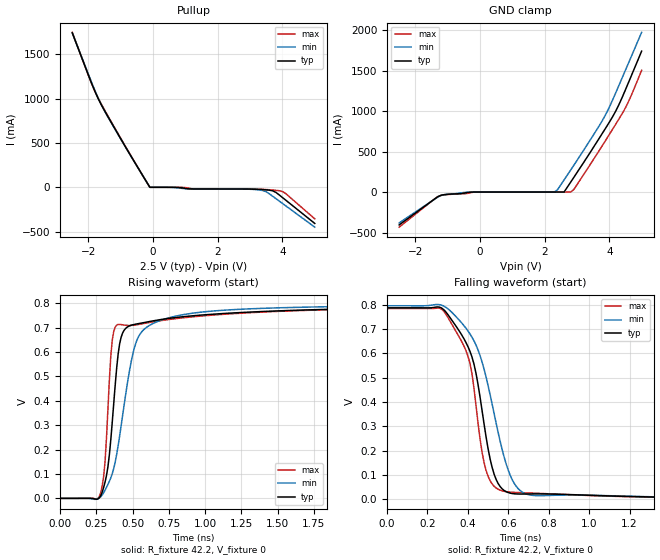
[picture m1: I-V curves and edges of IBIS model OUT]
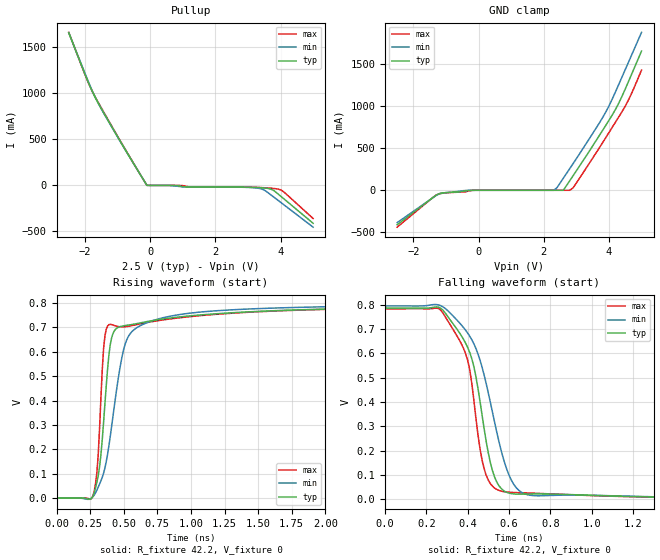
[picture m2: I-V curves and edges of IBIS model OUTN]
|   IBIS File of SG2520HHN D
|   HCSL Zdiff=85, Vcc=2.5V, fo>212.5MHz
[IBIS Ver]   3.2
[File Name]   sg2520hhn_hf_85_25v.ibs
[File Rev]   1.0
[Date]   Aug. 4, 2020
[Source]
[Notes]
Created by Minoru Kozaki
[Disclaimer]
Seiko Epson Corporation makes no warranty with respect to the
information contained herein.
[Copyright]
Copyright(C) 2020, Seiko Epson Corporation. All rights reserved.
|   Component
[Component]   SG2520HHN
[Manufacturer]  Seiko Epson Corporation
[Package]
R_pkg   17.7m   NA   NA
L_pkg   235p   NA   NA
C_pkg   208f   NA   NA
[Pin]   signal_name   model_name   R_pin   L_pin   C_pin
1   OE/ST   NC
2   NC   NC
3   GND   GND
4   OUT   OUT   17.7m   235p   208f
5   OUTN   OUTN   10.4m   129p   221f
6   VCC   POWER
[Diff Pin] inv_pin  vdiff  tdelay_typ
4   5   0   0
| Models and submodels in the file (2): OUT (Open_source), OUTN (Open_source)
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|   Model OUT
[Model]   OUT
Model_type   Open_source
Polarity   Non-Inverting
Vref = 0
Vmeas = 0.4
Rref = 42.2
Cref = 0
C_comp   12.0p   12.0p   12.0p
[Temperature Range]   25   105   -40
[Voltage Range]   2.5   2.25   2.75
[Pullup Reference]   2.5   2.25   2.75
[GND Clamp Reference]   0   0   0
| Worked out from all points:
|   GND clamp passes 1 mA (typ) near -0.25 V on its own axis
|   falling waveform, R_fixture 42.2, V_fixture 0: 20-80 % time 113ps typ, 146ps min, 96.9ps max; typ from 0.787 V to 0 V
|   rising waveform, R_fixture 42.2, V_fixture 0: 20-80 % time 74ps typ, 139ps min, 45.8ps max; typ from 0 V to 0.786 V
[Pullup]
-2.5V     1.74A      1.738A     1.746A
-1.9V     1.169A     1.18A      1.166A
-1.7V     1A         1.006A     1.004A
-1.3V     734.6mA    730.6mA    742.7mA
-100mV    31.32uA    15.33uA    89.15uA
700mV     -480.9uA   -4.431mA   -3.81uA
1.1V      -17.61mA   -18.31mA   -9.992mA
2.9V      -19.54mA   -20.86mA   -19.1mA
3.4V      -25.62mA   -36.48mA   -23.79mA
3.7V      -39.9mA    -101.2mA   -30.43mA
4V        -114.7mA   -181.3mA   -47.79mA
5V        -407mA     -448.8mA   -355mA
[GND Clamp]
-2.5V     -405.6mA   -380.9mA   -433.4mA
-1.2V     -39.03mA   -41.71mA   -40.52mA
-100mV    -21.28uA   -12.94uA   -96.75uA
2.3V      -1.475uA   3.582uA    -3.007uA
2.4V      -1.333uA   29.72mA    -2.745uA
2.6V      31.32uA    149mA      -2.258uA
2.8V      119.4mA    268.7mA    13.29uA
2.9V      179.5mA    328.8mA    29.86mA
3.8V      734.6mA    893.4mA    583.2mA
4.2V      1A         1.226A     838.7mA
4.6V      1.358A     1.598A     1.122A
5V        1.74A      1.972A     1.502A
[Falling Waveform]
R_fixture = 42.2
V_fixture = 0
V_fixture_min = 0
V_fixture_max = 0
0s        786.9mV    795.4mV    783.9mV
270ps     786.1mV    797.8mV    781.5mV
400ps     628.6mV    692.7mV    589.6mV
440ps     519.3mV    634.7mV    388.3mV
470ps     366.9mV    565.6mV    195.5mV
490ps     257.5mV    503.4mV    119.6mV
540ps     81.7mV     313mV      46.71mV
610ps     25.54mV    98.18mV    29.88mV
740ps     22.51mV    15.47mV    25.17mV
4ns       226uV      311uV      200uV
[Rising Waveform]
R_fixture = 42.2
V_fixture = 0
V_fixture_min = 0
V_fixture_max = 0
0s        91uV       119uV      90uV
280ps     10.98mV    6.696mV    24.03mV
310ps     67.4mV     33.71mV    153mV
340ps     181.4mV    70.52mV    490.8mV
360ps     316.4mV    102.1mV    650.3mV
400ps     591.3mV    215.8mV    712.6mV
440ps     687.8mV    377.4mV    710.3mV
530ps     714.9mV    649mV      711.6mV
750ps     737.5mV    739.9mV    733mV
4ns       786mV      794.4mV    783.4mV
[Ramp]
R_load = 42.2
dV/dt_r   0.47399/74.27p   0.47770/139.24p   0.47299/45.61p
dV/dt_f   0.47399/114.27p   0.47770/145.79p   0.47299/98.44p
|   Model OUTN
[Model]   OUTN
Model_type   Open_source
Polarity   Inverting
Vref = 0
Vmeas = 0.4
Rref = 42.2
Cref = 0
C_comp   12.0p   12.0p   12.0p
[Temperature Range]   25   105   -40
[Voltage Range]   2.5   2.25   2.75
[Pullup Reference]   2.5   2.25   2.75
[GND Clamp Reference]   0   0   0
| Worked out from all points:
|   GND clamp passes 1 mA (typ) near -0.25 V on its own axis
|   falling waveform, R_fixture 42.2, V_fixture 0: 20-80 % time 111ps typ, 144ps min, 94.5ps max; typ from 0.786 V to 0 V
|   rising waveform, R_fixture 42.2, V_fixture 0: 20-80 % time 73.6ps typ, 140ps min, 45.4ps max; typ from 0 V to 0.785 V
[Pullup]
-2.5V     1.655A     1.656A     1.659A
-2V       1.203A     1.213A     1.2A
-1.7V     961mA      964.5mA    966.5mA
-1.2V     648.2mA    644.8mA    655mA
-100mV    31.32uA    15.33uA    89.16uA
700mV     -480.7uA   -4.424mA   -3.81uA
1.1V      -17.6mA    -18.3mA    -9.944mA
2.9V      -19.54mA   -20.85mA   -19.1mA
3.4V      -25.62mA   -36.45mA   -23.78mA
3.7V      -39.89mA   -101.8mA   -30.43mA
4V        -115.5mA   -182.6mA   -47.85mA
5V        -411.2mA   -453mA     -359mA
[GND Clamp]
-2.5V     -409.8mA   -384.4mA   -438.4mA
-1.2V     -39.02mA   -41.69mA   -40.54mA
-100mV    -21.28uA   -12.94uA   -96.74uA
2.3V      -1.475uA   3.582uA    -3.007uA
2.4V      -1.333uA   28.69mA    -2.745uA
2.6V      31.32uA    143.8mA    -2.258uA
2.8V      115.3mA    259.4mA    13.29uA
2.9V      173.3mA    317.4mA    28.82mA
3.9V      770mA      928.3mA    624.2mA
4.2V      961mA      1.17A      809.3mA
4.5V      1.203A     1.434A     1A
5V        1.655A     1.878A     1.429A
[Falling Waveform]
R_fixture = 42.2
V_fixture = 0
V_fixture_min = 0
V_fixture_max = 0
0s        786.2mV    794.7mV    783.2mV
260ps     789.2mV    798.7mV    783.6mV
360ps     684.8mV    725.7mV    654.3mV
400ps     624.1mV    683.3mV    571.4mV
430ps     545.3mV    639.2mV    406.9mV
490ps     236.1mV    474.3mV    98.33mV
540ps     72.58mV    279.3mV    41.25mV
600ps     25.8mV     99.63mV    29.37mV
730ps     22.21mV    15mV       25.04mV
4ns       223uV      303uV      197uV
[Rising Waveform]
R_fixture = 42.2
V_fixture = 0
V_fixture_min = 0
V_fixture_max = 0
0s        86uV       124uV      89uV
270ps     7.717mV    5.201mV    8.364mV
290ps     41.3mV     21.54mV    58.77mV
310ps     91.7mV     45.04mV    176.4mV
350ps     310.2mV    102.3mV    611.9mV
390ps     587.9mV    215.6mV    711.1mV
430ps     685.5mV    377mV      707.2mV
520ps     708mV      645.6mV    703.1mV
750ps     730.9mV    733mV      727mV
4ns       785.3mV    793.6mV    782.5mV
[Ramp]
R_load = 42.2
dV/dt_r   0.47393/74.02p   0.47765/140.84p   0.47292/45.15p
dV/dt_f   0.47393/112.11p   0.47765/144.30p   0.47292/96.19p
